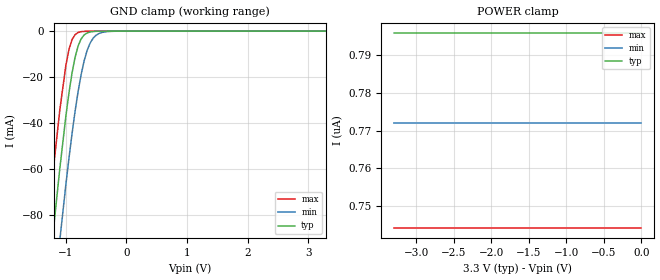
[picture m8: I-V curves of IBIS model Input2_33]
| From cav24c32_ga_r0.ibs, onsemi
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|//////////////////////////////////////////////////////////////////////////////
|//////////////////////////////////////////////////////////////////////////////
[Model]  Input2_33
Model_type Input
Vinh = 2.31
Vinl = 0.99
|  variable   typ   min   max
C_comp   6pF   6pF   6pF
|//////////////////////////////////////////////////////////////////////////////
[Temperature Range]   25   125   -40
|//////////////////////////////////////////////////////////////////////////////
[Voltage Range]   3.30V   3.00V   3.60V
|//////////////////////////////////////////////////////////////////////////////
[POWER Clamp Reference] 3.30V   3.00V   3.60V
|//////////////////////////////////////////////////////////////////////////////
[GND Clamp Reference]   0V   0V   0V
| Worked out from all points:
|   GND clamp passes 1 mA (typ) near -0.66 V on its own axis
|//////////////////////////////////////////////////////////////////////////////
[GND Clamp]
|   Voltage   I(typ)   I(min)   I(max)
-3.3V     -720mA     -745mA     -702mA
-1.3V     -111mA     -143mA     -84.7mA
-1.2V     -84.6mA    -116mA     -58.1mA
-1.1V     -59.4mA    -90.5mA    -34mA
-1V       -36.7mA    -66.4mA    -14.7mA
-950mV    -26.8mA    -55.2mA    -7.98mA
-900mV    -18.3mA    -44.7mA    -3.72mA
-800mV    -6.54mA    -26.4mA    -589uA
-650mV    -779uA     -8.39mA    -43uA
-550mV    -167uA     -3.05mA    -17.3uA
-400mV    -21.9uA    -543uA     -9.92uA
3.3V      796nA      772nA      744nA
|//////////////////////////////////////////////////////////////////////////////
[POWER Clamp]
|   Voltage   I(typ)   I(min)   I(max)
-3.3V     796nA      772nA      744nA
-3.2V     796nA      772nA      744nA
-3.1V     796nA      772nA      744nA
0V        796nA      772nA      744nA
